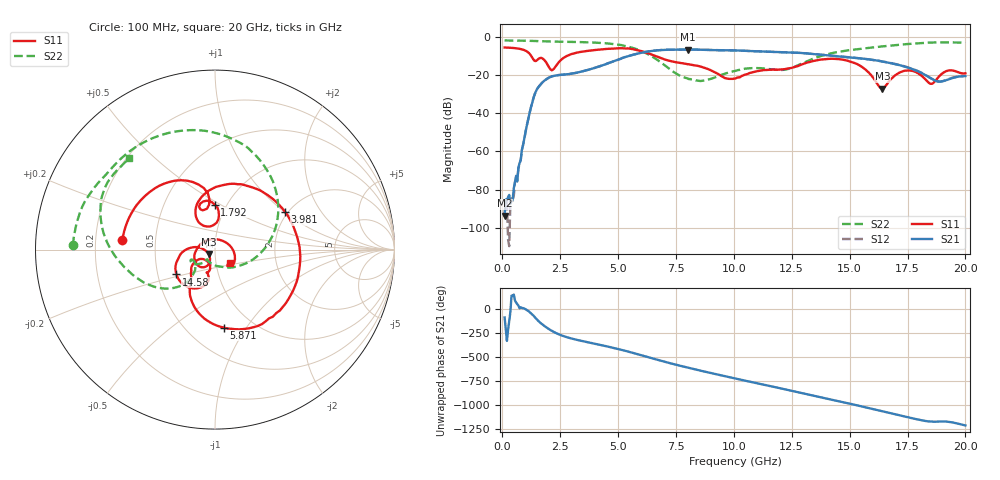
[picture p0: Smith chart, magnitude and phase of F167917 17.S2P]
!  2-Port S-parameters saved by WinCal
! VAR MeasName=S-Parameters (CALIBRATED_DATA) read from VNA (N5242A)
! VAR MeasDate=2016-11-22 9:00:34
! VAR NAME=F167917 17
! VAR FILENAME=F167917 17.S2P
! VAR DATE=2016-11-22 9:00:34
! VAR PHYS_PORTS=1,2
# Hz S DB R 50
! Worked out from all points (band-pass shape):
!   401 points, 100 MHz to 20 GHz, reference 50 ohm
!   highest |S21| = -6.78 dB at 8.01 GHz (marker M1); lowest = -93.7 dB at 100 MHz (marker M2)
!   |S21| within 3 dB of the highest: 5.572 GHz to 14.02 GHz (8.447 GHz wide, 86.2 % of centre)
!   lowest |S11| = -27.2 dB at 16.42 GHz (marker M3), VSWR 1.09, Z = 46.5 - j2.31 ohm
!   |S11| at or under -10 dB: 1.243 GHz to 2.814 GHz (1.571 GHz wide, 77.5 % of centre); 6.584 GHz to end of sweep
!   |S22| runs from -23.2 to -2.0 dB; largest |S21 - S12| = 0.0042
!   S11 on the Smith chart (normalised r, x): 100 MHz: 0.32, +0.05; 1.792 GHz: 0.88, +0.47; 3.981 GHz: 1.94, +1.01; 5.871 GHz: 0.74, -0.79; 14.58 GHz: 0.63, -0.19; 20 GHz: 1.16, -0.17
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1e8  -5.71 174.2  -93.66 -92.4  -92.41 38.6  -2.02 178.3
5.4775e8  -6.06 147.4  -76.14 84.1  -76.14 65.3  -2.09 171.1
1.294e9  -11.04 96.3  -34.62 -60.8  -34.59 -60.9  -2.26 159.0
1.7915e9  -12.01 90.3  -23.32 -176.3  -23.30 -176.4  -2.47 151.3
2.13975e9  -17.63 101.9  -20.86 128.9  -20.82 128.7  -2.63 146.1
3.43325e9  -7.95 61.4  -18.27 23.6  -18.27 23.4  -2.90 123.0
3.9805e9  -7.06 28.2  -16.41 -4.8  -16.41 -4.9  -3.14 110.2
4.876e9  -6.19 -25.0  -12.67 -52.6  -12.66 -52.5  -4.01 83.1
5.871e9  -7.19 -83.8  -8.85 -115.3  -8.81 -115.2  -6.88 39.9
6.7665e9  -10.85 -119.2  -7.11 -176.0  -7.09 -176.0  -12.80 -11.4
8.01025e9  -14.45 -134.7  -6.78 107.2  -6.75 107.1  -21.93 -105.7
1.005e10  -21.94 -117.6  -7.28 -5.0  -7.28 -5.0  -17.99 -140.3
1.1642e10  -17.29 -109.6  -7.95 -88.6  -7.93 -88.5  -17.12 -156.4
1.338325e10  -12.92 -111.0  -9.05 177.7  -9.02 178.0  -11.77 -131.9
1.457725e10  -11.86 -147.2  -10.41 115.1  -10.35 115.2  -7.88 -149.8
1.55225e10  -15.77 -179.7  -11.51 64.6  -11.49 64.5  -6.30 -163.9
1.6418e10  -27.22 -145.2  -13.08 13.8  -12.98 14.3  -5.13 -175.6
1.67165e10  -23.26 -114.3  -13.69 -3.2  -13.70 -2.6  -4.77 -179.6
1.746275e10  -17.73 -136.7  -16.02 -45.6  -15.89 -44.9  -3.93 170.0
1.85075e10  -24.71 90.8  -21.82 -93.7  -21.77 -93.6  -3.12 153.8
1.8806e10  -21.64 18.3  -23.49 -94.5  -23.36 -93.6  -3.03 148.8
2e10  -19.21 -42.1  -20.66 -133.6  -20.52 -133.4  -3.12 133.1
